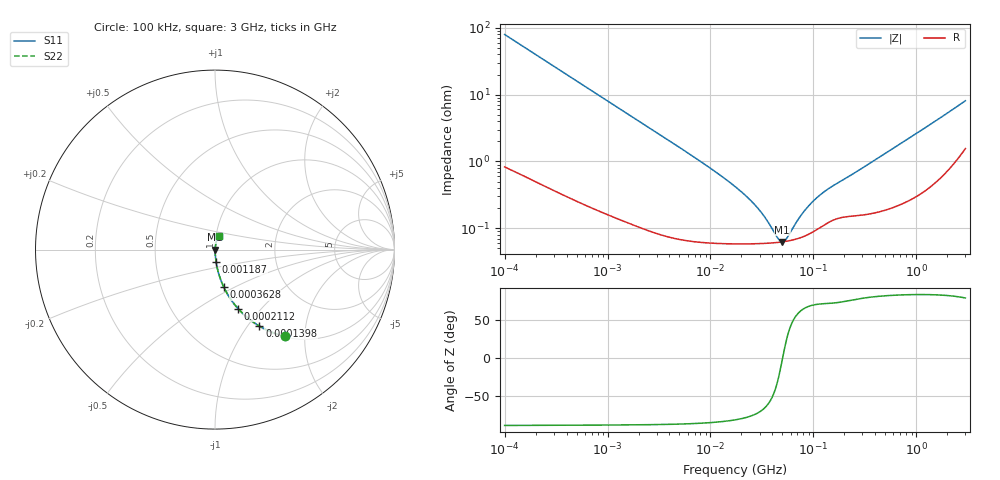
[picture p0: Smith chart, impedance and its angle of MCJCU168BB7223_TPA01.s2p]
! MCJCU168BB7223_TPA01  S-PARAMETER MODEL  ( Standard Model )
! Model Generated by TAIYO YUDEN Corporation (http://www.ty-top.com)
! Version 1.0
! TAIYO YUDEN Control No. 220601
! Copyright(c) 2015 TAIYO YUDEN CO.,LTD. All Rights Reserved.
! Product Description (link to TY-COMPAS)
! https://ds.yuden.co.jp/TYCOMPAS/or/detail?pn=MCJCU168BB7223KTPA01&u=M
! Products Name : Multilayer Ceramic Capacitors
! Characteristics :
!  Capacitance : 0.022 [uF] , Rated Voltage : 50 [V] , TCC : X7R
!  Case Size : 1.6 x 0.8 / 0.063 x 0.031 [mm/inch] , Thickness : 0.8 / 0.031 [mm/inch]
!  (Conditions: Temperature = 25 [degC] , DC Bias Voltage = 0 [V])
! External Node Assignments :
!  1  o---| |---o  2
! GND o---------o GND
! Frequency Range : 100kHz  -  3GHz  [ 401 STEP ]
# MHZ S RI R 50
! Freq[MHz].  S11 Real  S11 Imag  S21 Real  S21 Imag  S12 Real  S12 Imag  S22 Real  S22 Imag
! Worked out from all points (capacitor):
!   401 points, 100 kHz to 3 GHz, reference 50 ohm
!   read as one part in series: C = 20 nF near 105.3 kHz
!   lowest |Z| = 62.8 mohm at 49.83 MHz (marker M1)
!   series resonance near 50.3 MHz, so ESL is about 500 pH
!   S11 on the Smith chart (normalised r, x): 100 kHz: 1.02, -1.59; 139.8 kHz: 1.01, -1.14; 211.2 kHz: 1.01, -0.76; 362.8 kHz: 1.01, -0.44; 1.187 MHz: 1.00, -0.14; 3 GHz: 1.03, +0.16
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0.1  0.3884 -0.4822  0.6116 0.4822  0.6116 0.4822  0.3884 -0.4822
0.1398  0.2477 -0.426  0.7523 0.426  0.7523 0.426  0.2477 -0.426
0.21115  0.1284 -0.3283  0.8716 0.3283  0.8716 0.3283  0.1284 -0.3283
0.362777  0.0494 -0.2096  0.9506 0.2096  0.9506 0.2096  0.0494 -0.2096
0.562235  0.0223 -0.1397  0.9777 0.1397  0.9777 0.1397  0.0223 -0.1397
1.18716  0.00605 -0.0678  0.9939 0.0678  0.9939 0.0678  0.00605 -0.0678
3.161081  0.00148 -0.0257  0.9985 0.0257  0.9985 0.0257  0.00148 -0.0257
9.331111  0.000677 -0.00849  0.9993 0.00849  0.9993 0.00849  0.000677 -0.00849
17.7727  0.000601 -0.00405  0.9994 0.00405  0.9994 0.00405  0.000601 -0.00405
23.59795  0.000592 -0.00272  0.9994 0.00272  0.9994 0.00272  0.000592 -0.00272
29.00125  0.000593 -0.00189  0.9994 0.00189  0.9994 0.00189  0.000593 -0.00189
34.73492  0.000598 -0.00124  0.9994 0.00124  0.9994 0.00124  0.000598 -0.00124
44.94634  0.000615 -0.00037  0.9994 0.00037  0.9994 0.00037  0.000615 -0.00037
49.82709  0.000627 -3.1e-05  0.9994 3.1e-05  0.9994 3.1e-05  0.000627 -3.1e-05
52.46276  0.000634 0.000138  0.9994 -0.000138  0.9994 -0.000138  0.000634 0.000138
55.23785  0.000642 0.000308  0.9994 -0.000308  0.9994 -0.000308  0.000642 0.000308
75.25761  0.000727 0.00136  0.9993 -0.00136  0.9993 -0.00136  0.000727 0.00136
97.38194  0.000875 0.0023  0.9991 -0.0023  0.9991 -0.0023  0.000875 0.0023
143.341  0.00126 0.0038  0.9987 -0.0038  0.9987 -0.0038  0.00126 0.0038
547.5153  0.00216 0.0143  0.9978 -0.0143  0.9978 -0.0143  0.00216 0.0143
1420.79  0.00569 0.0367  0.9943 -0.0367  0.9943 -0.0367  0.00569 0.0367
3000  0.0214 0.0767  0.9786 -0.0767  0.9786 -0.0767  0.0214 0.0767
